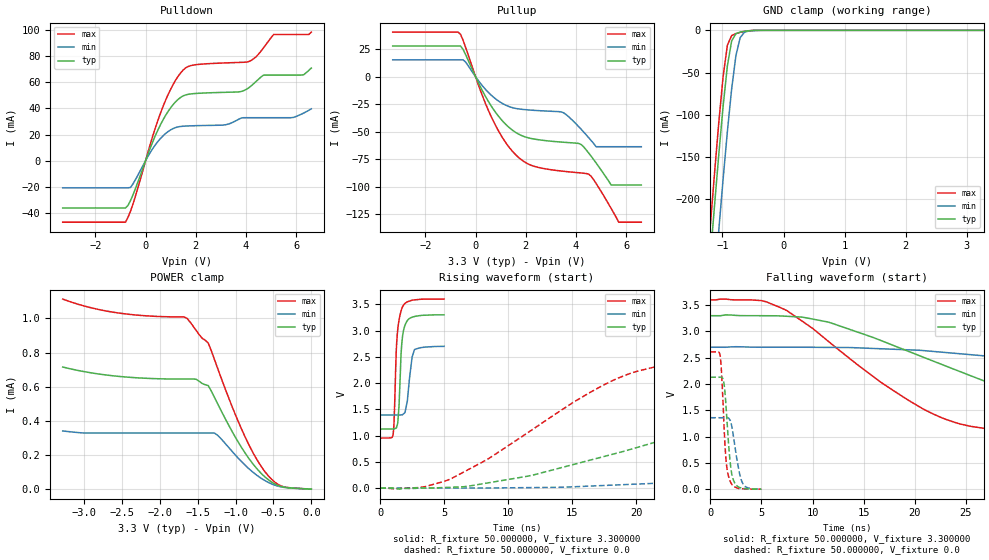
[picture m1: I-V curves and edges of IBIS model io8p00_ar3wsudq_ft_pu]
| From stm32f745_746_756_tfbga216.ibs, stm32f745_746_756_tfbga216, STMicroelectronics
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|   Model io8p00_ar3wsudq_ft_pu
[Model]  io8p00_ar3wsudq_ft_pu
Model_type I/O
Polarity   Non-Inverting
Enable   Active-Low
Vinl =   0.990000V
Vinh =   2.310000V
Vmeas =  1.650000V
Cref =   50.000000pF
Rref =   100.000000M
Vref =   0.0V
C_comp   3.843200pF   3.761700pF   3.937000pF
[Temperature Range]   25.000000   0.125000k   -40.000000
[Pullup Reference]   3.300000V   2.700000V   3.600000V
[Pulldown Reference]   0.0V   0.0V   0.0V
[POWER Clamp Reference]   3.300000V   2.700000V   3.600000V
[GND Clamp Reference]   0.0V   0.0V   0.0V
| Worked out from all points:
|   slope of the pulldown table from 0 to 0.495 V, typ, clamps not added: 20.9 ohm
|   slope of the pullup table from 0 to 0.495 V, typ, clamps not added: 22.6 ohm
|   GND clamp passes 1 mA (typ) near -0.62 V on its own axis
|   rising waveform, R_fixture 50.000000, V_fixture 3.300000: 20-80 % time 267ps typ, 350ps min, 280ps max; typ from 1.12 V to 3.3 V
|   rising waveform, R_fixture 50.000000, V_fixture 0.0: 20-80 % time 19.7ns typ, 50.7ns min, 10.4ns max; typ from 0.001 V to 2.13 V
|   falling waveform, R_fixture 50.000000, V_fixture 3.300000: 20-80 % time 18.5ns typ, 38.5ns min, 11.3ns max; typ from 3.3 V to 1.12 V
|   falling waveform, R_fixture 50.000000, V_fixture 0.0: 20-80 % time 504ps typ, 695ps min, 423ps max; typ from 2.13 V to 0.001 V
[Pulldown]
|Voltage   I(typ)   I(min)   I(max)
-3.3V     -36.18mA   -20.77mA   -47.07mA
-800mV    -36.18mA   -20.77mA   -47.07mA
-600mV    -30.5mA    -20.52mA   -38.69mA
700mV     31.4mA     19.11mA    41.71mA
1.2V      45.15mA    25.37mA    61.75mA
1.6V      50.35mA    26.5mA     71.06mA
3.1V      52.28mA    27.26mA    74.76mA
4.1V      55.65mA    32.89mA    75.79mA
4.7V      65.5mA     32.89mA    86.49mA
5.1V      65.5mA     32.89mA    96.55mA
6.3V      65.83mA    36.49mA    96.55mA
6.6V      70.88mA    39.7mA     98.4mA
[Pullup]
|Voltage   I(typ)   I(min)   I(max)
-3.3V     28mA       15.42mA    40.61mA
-700mV    28mA       15.42mA    40.61mA
-400mV    20.3mA     13.47mA    26.92mA
600mV     -25.77mA   -16.23mA   -35.13mA
1.6V      -50.64mA   -28.8mA    -70.96mA
3.5V      -59.52mA   -32.72mA   -85.91mA
4.2V      -61.52mA   -47.61mA   -87.45mA
4.5V      -69.2mA    -55.26mA   -88.43mA
4.8V      -78.36mA   -63.6mA    -97mA
5.4V      -98.4mA    -63.6mA    -119.7mA
5.7V      -98.4mA    -63.6mA    -132.2mA
6.6V      -98.4mA    -63.6mA    -132.2mA
[GND_clamp]
|Voltage   I(typ)   I(min)   I(max)
-3.3V     -2.328A    -2.406A    -2.303A
-1.2V     -270.2mA   -361.4mA   -232.1mA
-1.13V    -207.3mA   -298.1mA   -169mA
-1.06V    -146.7mA   -236.2mA   -108.8mA
-990mV    -90.18mA   -176.4mA   -54.96mA
-920mV    -42.21mA   -120mA     -17.68mA
-850mV    -12.57mA   -69.47mA   -6.265mA
-780mV    -3.971mA   -30.01mA   -3.886mA
-710mV    -2.1mA     -8.615mA   -2.382mA
-640mV    -1.148mA   -2.283mA   -1.22mA
-570mV    -524uA     -821.5uA   -476.8uA
3.28V     0A         0A         0A
[POWER_clamp]
|Voltage   I(typ)   I(min)   I(max)
-3.28V    715.1uA    340.8uA    1.113mA
-2.6V     662.9uA    328.8uA    1.035mA
-1.64V    645uA      328.8uA    1mA
-1.52V    643.3uA    328.8uA    929.5uA
-1.36V    606.3uA    328.8uA    855.6uA
-1.24V    503.7uA    316.8uA    712.3uA
-960mV    272.5uA    179.4uA    391.9uA
-800mV    165.1uA    110.4uA    239.2uA
-640mV    83.2uA     57.57uA    119.3uA
-520mV    40.52uA    29.83uA    56.09uA
-400mV    15.54uA    13.29uA    18.7uA
0V        0A         0A         0A
[Ramp]
| variable   typ   min   max
dV/dt_r  1.27711/19.71979n   0.81591/50.81131n   1.56688/10.34235n
dV/dt_f  1.30656/18.47745n   0.78402/38.54083n   1.58713/11.31959n
R_load = 50.000000
[Rising Waveform]
R_fixture= 50.000000
V_fixture= 3.300000
V_fixture_min= 2.700000
V_fixture_max= 3.600000
|time   V(typ)   V(min)   V(max)
0s        1.125V     1.393V     954.7mV
1.001ns   1.127V     1.393V     1.008V
1.071ns   1.128V     1.393V     1.225V
1.331ns   1.209V     1.393V     2.937V
1.461ns   1.555V     1.392V     3.19V
1.632ns   2.577V     1.394V     3.378V
1.732ns   2.871V     1.398V     3.447V
2.112ns   3.188V     1.657V     3.548V
2.673ns   3.267V     2.637V     3.584V
4.985ns   3.3V       2.7V       3.6V
[Rising Waveform]
R_fixture= 50.000000
V_fixture= 0.0
V_fixture_min= 0.0
V_fixture_max= 0.0
|time   V(typ)   V(min)   V(max)
0s        1.088mV    1.043mV    1.136mV
5.506ns   17.34mV    2.784mV    175.3mV
11.51ns   227.6mV    10.66mV    1.053V
19.52ns   735.5mV    72.25mV    2.183V
27.03ns   1.261V     157.8mV    2.478V
38.54ns   1.853V     360.8mV    2.575V
57.56ns   2.069V     711.2mV    2.608V
88.09ns   2.119V     1.133V     2.613V
115.1ns   2.128V     1.293V     2.613V
249.2ns   2.13V      1.36V      2.613V
[Falling Waveform]
R_fixture= 50.000000
V_fixture= 3.300000
V_fixture_min= 2.700000
V_fixture_max= 3.600000
|time   V(typ)   V(min)   V(max)
0s        3.3V       2.7V       3.6V
5.506ns   3.299V     2.7V       3.562V
11.51ns   3.18V      2.697V     2.818V
22.02ns   2.42V      2.617V     1.412V
31.03ns   1.758V     2.448V     1.082V
38.54ns   1.42V      2.267V     1.023V
45.55ns   1.288V     2.095V     1.002V
63.56ns   1.185V     1.729V     970.7mV
86.59ns   1.146V     1.528V     958.1mV
249.2ns   1.125V     1.393V     954.7mV
[Falling Waveform]
R_fixture= 50.000000
V_fixture= 0.0
V_fixture_min= 0.0
V_fixture_max= 0.0
|time   V(typ)   V(min)   V(max)
0s        2.13V      1.36V      2.613V
981ps     2.131V     1.36V      2.52V
1.151ns   2.122V     1.359V     2.039V
1.311ns   2.041V     1.359V     1.353V
1.522ns   1.635V     1.361V     598.3mV
1.902ns   597.9mV    1.322V     173.8mV
2.292ns   159mV      969.8mV    54.18mV
2.853ns   34.43mV    304.7mV    13.43mV
3.173ns   16.52mV    111.3mV    9.01mV
4.985ns   1.088mV    1.043mV    1.136mV
